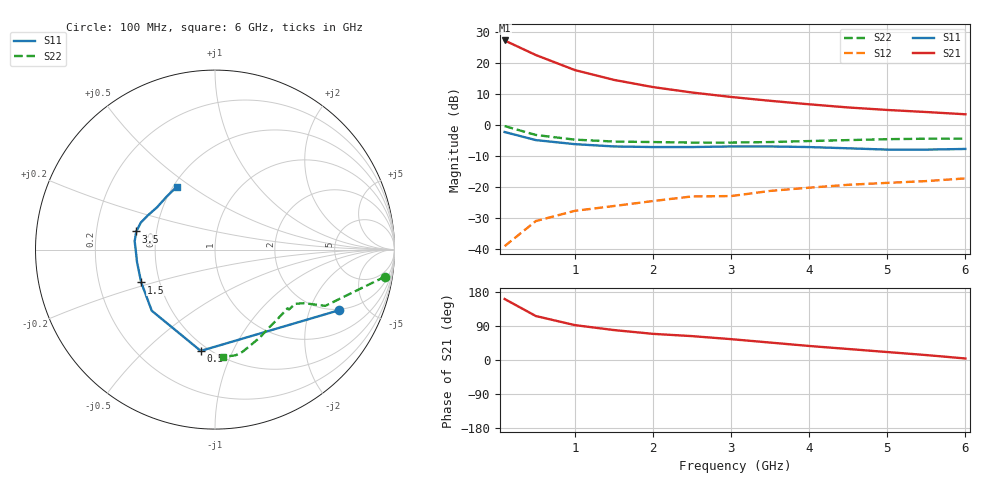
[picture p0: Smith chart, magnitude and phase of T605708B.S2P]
!AT-60570
!S-PARAMETERS at Vce=8V  Ic=10mA.  LAST UPDATED 07-21-92
# ghz s ma r 50
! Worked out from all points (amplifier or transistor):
!   13 points, 100 MHz to 6 GHz, reference 50 ohm
!   highest |S21| = 27.3 dB at 100 MHz (marker M1)
!   |S21| within 3 dB of that: start of sweep to 354.5 MHz
!   unconditionally stable (mu >= 1): 1.429 GHz to end of sweep
!   at 1 GHz: K = 0.80, MSG = 22.7 dB, |S12| = -27.7 dB
!   at 3 GHz: K = 1.32, MAG = 12.6 dB, |S12| = -23.0 dB
!   at 6 GHz: K = 1.16, MAG = 7.9 dB, |S12| = -17.3 dB
!   S11 on the Smith chart (normalised r, x): 100 MHz: 1.95, -3.23; 500 MHz: 0.46, -0.76; 1.5 GHz: 0.39, -0.18; 3.5 GHz: 0.38, +0.10; 6 GHz: 0.52, +0.44
0.1  0.77 -26.0  23.25 161.0  0.011 79.0  0.96 -9.0
0.5  0.57 -98.0  13.51 116.0  0.028 49.0  0.69 -27.0
1  0.49 -136.0  7.72 92.0  0.041 45.0  0.58 -31.0
1.5  0.45 -156.0  5.36 79.0  0.049 45.0  0.54 -34.0
2  0.44 -171.0  4.1 69.0  0.059 48.0  0.53 -39.0
2.5  0.44 -177.0  3.35 63.0  0.07 51.0  0.52 -39.0
3  0.45 174.0  2.84 55.0  0.071 52.0  0.52 -47.0
3.5  0.45 167.0  2.46 46.0  0.086 52.0  0.53 -56.0
4  0.44 160.0  2.16 37.0  0.097 50.0  0.55 -63.0
4.5  0.42 153.0  1.92 29.0  0.108 47.0  0.57 -70.0
5  0.4 144.0  1.75 21.0  0.116 44.0  0.59 -75.0
5.5  0.4 132.0  1.62 13.0  0.124 41.0  0.6 -79.0
6  0.41 121.0  1.49 4.0  0.137 38.0  0.6 -86.0
